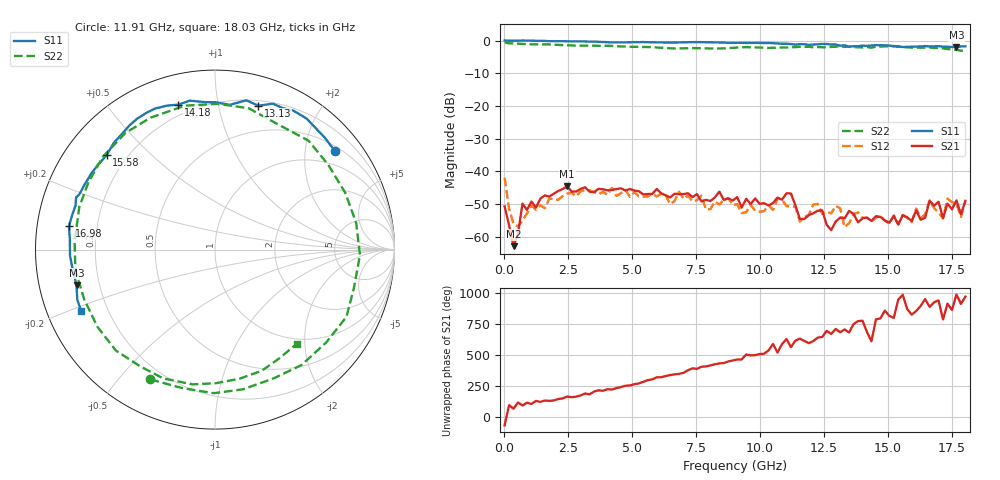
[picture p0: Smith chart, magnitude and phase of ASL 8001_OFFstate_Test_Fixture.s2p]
!ASL 8001 Wideband SPST Switch
!OFF State Test Fixture S-parameter data from 10MHz-18 GHz
!Agilent Technologies,N5230A,MY45000142,A.04.83
!Agilent N5230A: A.04.83
!Date: Tuesday, December 12, 2006 14:29:38
!Correction: S11(Full 2 Port SOLT,1,2) S21(Full 2 Port SOLT,1,2) S12(Full 2 Port SOLT,1,2) S22(Full 2 Port SOLT,1,2)
!S2P File: Measurements: S11, S21, S12, S22:
# Hz S  dB  R 50
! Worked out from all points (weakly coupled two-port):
!   104 points, 10 MHz to 18.03 GHz, reference 50 ohm
!   highest |S21| = -44.65 dB at 2.459 GHz (marker M1); lowest = -63.0 dB at 359.9 MHz (marker M2)
!   lowest |S11| = -2.0 dB at 17.68 GHz (marker M3), VSWR 8.82, Z = 5.76 - j6.2 ohm
!   |S11| at or under -10 dB: nowhere
!   |S22| runs from -3.2 to -0.6 dB; largest |S21 - S12| = 0.011
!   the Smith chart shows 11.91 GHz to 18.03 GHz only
!   S11 on the Smith chart (normalised r, x): 11.91 GHz: 0.62, +2.68; 13.13 GHz: 0.25, +1.32; 14.18 GHz: 0.15, +0.77; 15.58 GHz: 0.13, +0.37; 16.98 GHz: 0.10, +0.08; 18.03 GHz: 0.10, -0.22
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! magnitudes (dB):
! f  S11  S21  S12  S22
! 10 MHz  0.1  -50.8  -42.0  -0.6
! 359.9 MHz  0.0  -63.0  -56.1  -0.8
! 709.8 MHz  0.1  -49.9  -55.0  -1.0
! 2.459 GHz  -0.2  -44.6  -46.8  -1.4
! 3.159 GHz  -0.2  -44.9  -45.7  -1.5
! 6.133 GHz  -0.5  -46.7  -46.8  -2.2
! 9.107 GHz  -0.6  -47.9  -50.1  -2.1
! 11.21 GHz  -1.0  -46.8  -50.8  -2.0
! 11.56 GHz  -1.0  -54.6  -55.4  -1.9
! 11.91 GHz  -1.3  -53.4  -53.3  -1.9
! 12.08 GHz  -1.2  -52.9  -50.2  -2.0
! 13.13 GHz  -1.5  -54.2  -51.4  -1.7
! 13.31 GHz  -1.4  -54.5  -57.1  -1.9
! 14.18 GHz  -1.6  -54.2  -54.3  -1.9
! 15.06 GHz  -1.5  -55.8  -56.0  -1.7
! 15.58 GHz  -1.9  -53.5  -53.4  -2.0
! 16.98 GHz  -1.7  -49.4  -52.7  -2.2
! 17.16 GHz  -1.8  -54.4  -54.4  -2.4
! 17.33 GHz  -1.8  -49.9  -48.4  -2.6
! 17.68 GHz  -2.0  -48.9  -49.9  -2.8
! 17.85 GHz  -1.8  -53.2  -54.0  -3.1
! 18.03 GHz  -1.7  -49.0  -49.0  -3.2
